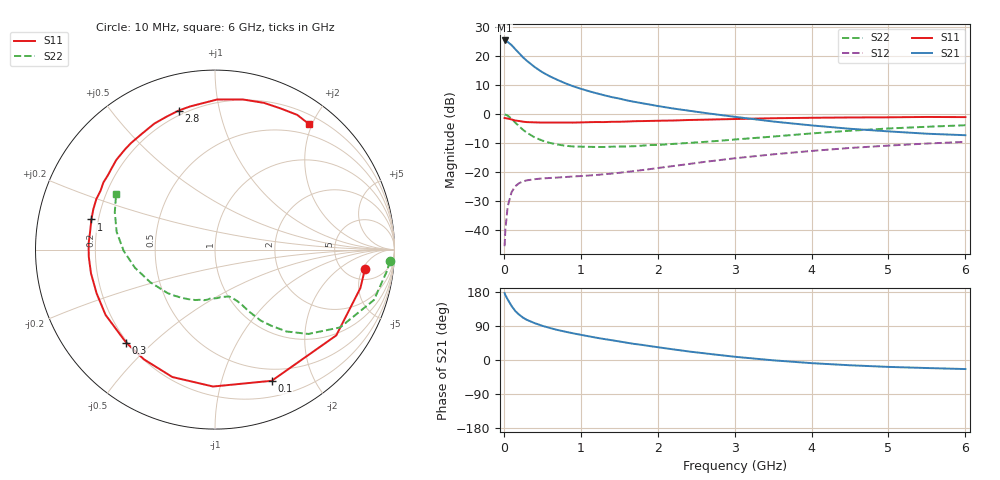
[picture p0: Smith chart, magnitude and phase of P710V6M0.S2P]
! SIEMENS Small Signal Semiconductors
! BFP196
! Si NPN RF Bipolar Junction Transistor in SOT143
! VCE = 10 V  IC = 6 mA
! Common Emitter S-Parameters:  May  1996
# GHz  S  MA  R  50
!  f  S11  S21  S12  S22
! GHz  MAG  ANG  MAG  ANG  MAG  ANG  MAG  ANG
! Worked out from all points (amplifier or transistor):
!   36 points, 10 MHz to 6 GHz, reference 50 ohm
!   highest |S21| = 25.3 dB at 10 MHz (marker M1)
!   |S21| within 3 dB of that: start of sweep to 148.7 MHz
!   unconditionally stable (mu >= 1): 1.117 GHz to 3.277 GHz
!   at 250 MHz: K = 0.28, MSG = 21.4 dB, |S12| = -23.3 dB
!   at 1.4 GHz: K = 1.13, MAG = 11.0 dB, |S12| = -20.7 dB
!   at 6 GHz: K = 0.98, MSG = 1.1 dB, |S12| = -9.7 dB
!   S11 on the Smith chart (normalised r, x): 10 MHz: 7.39, -5.59; 100 MHz: 0.37, -1.46; 300 MHz: 0.19, -0.41; 1 GHz: 0.17, +0.12; 2.8 GHz: 0.18, +0.76; 6 GHz: 0.33, +1.96
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0.01  0.8421 -7.5  18.34 176.7  0.0052 85.3  0.977 -3.8
0.02  0.838 -14.8  18.07 171.3  0.01 83.4  0.9649 -7.2
0.05  0.8276 -35.3  17.28 159.8  0.0252 71.6  0.9289 -17.6
0.1  0.7964 -66.6  15.29 142.7  0.0443 57.7  0.8205 -31.9
0.15  0.7629 -90.8  12.93 128.9  0.0564 46.9  0.701 -42.1
0.2  0.7487 -108.5  11.01 119.4  0.0636 39.8  0.6051 -48.9
0.25  0.7285 -122.9  9.365 111.7  0.0681 34.6  0.5265 -53.6
0.3  0.7168 -133.7  8.156 105.8  0.071 31.8  0.4707 -57.2
0.4  0.7101 -149.2  6.399 97.3  0.0743 27.8  0.3905 -61.4
0.5  0.7032 -159.8  5.198 90.3  0.0766 25.7  0.3441 -63.9
0.6  0.7035 -169.2  4.401 84.4  0.078 25.1  0.3137 -66.5
0.7  0.7043 -176.8  3.82 79.1  0.0794 25.4  0.2941 -69.0
0.8  0.7051 177.3  3.347 74.7  0.0809 25.7  0.2801 -71.3
1  0.7088 166.3  2.695 66.5  0.0841 27.4  0.2706 -75.4
1.1  0.7143 161.6  2.46 62.7  0.0859 28.6  0.2685 -78.3
1.6  0.7334 141.5  1.697 45.6  0.0995 35.0  0.2728 -93.2
2.2  0.7636 122.0  1.231 28.1  0.1252 39.1  0.3016 -111.3
2.8  0.8006 104.7  0.957 13.2  0.1583 38.5  0.3413 -131.1
3.5  0.8363 89.2  0.734 -0.8  0.1993 33.3  0.4038 -153.2
4.5  0.8619 71.5  0.55 -13.9  0.2568 23.0  0.5089 -179.2
5.5  0.8793 58.6  0.452 -21.2  0.3061 11.0  0.5957 159.6
6  0.8737 53.0  0.426 -23.9  0.3274 4.5  0.6329 150.5
